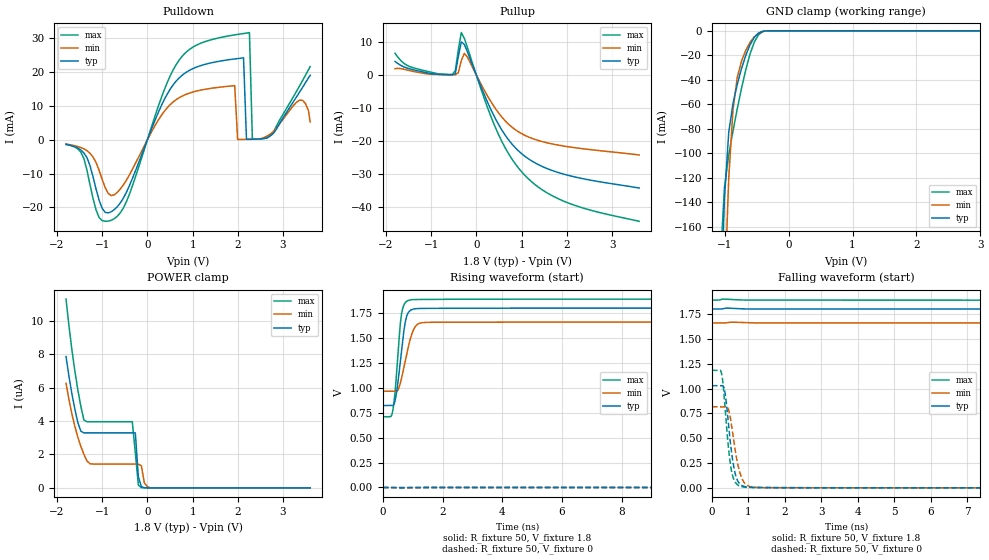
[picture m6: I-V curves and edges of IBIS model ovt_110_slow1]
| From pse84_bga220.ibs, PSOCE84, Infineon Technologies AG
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[Model] ovt_110_slow1
Model_type I/O
Enable   Active-High
Vinl  =  0.54
Vinh  =  1.26
Vmeas =  0.9
Cref  =  15e-12
| Capacitance   typ   min   max
C_comp   1.39974e-12   1.35992e-12   1.44753e-12
| Variables   typ   min   max
[GND Clamp Reference]   0   0   0
[POWER Clamp Reference]   1.8   1.66   1.89
[Pulldown Reference]   0   0   0
[Pullup Reference]   1.8   1.66   1.89
[Temperature Range]   25   125   -40
[Voltage Range]   1.8   1.66   1.89
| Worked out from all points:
|   slope of the pulldown table from 0 to 0.27 V, typ, clamps not added: 30.3 ohm
|   slope of the pullup table from 0 to 0.27 V, typ, clamps not added: 30.5 ohm
|   GND clamp passes 1 mA (typ) near -0.43 V on its own axis
|   falling waveform, R_fixture 50, V_fixture 1.8: 20-80 % time 92.1ns typ, 146ns min, 49.7ns max; typ from 1.8 V to 0.822 V
|   falling waveform, R_fixture 50, V_fixture 0: 20-80 % time 197ps typ, 231ps min, 178ps max; typ from 1.03 V to 0 V
|   rising waveform, R_fixture 50, V_fixture 1.8: 20-80 % time 231ps typ, 319ps min, 184ps max; typ from 0.822 V to 1.8 V
|   rising waveform, R_fixture 50, V_fixture 0: 20-80 % time 107ns typ, 168ns min, 63.3ns max; typ from 0 V to 1.03 V
[GND Clamp]
| Voltage   I(typ)   I(min)   I(max)
-1.271V   -717.5mA   -832.8mA   -643.6mA
-1.07V    -241.9mA   -348.3mA   -192.2mA
-1.003V   -137.2mA   -218.1mA   -128.1mA
-936.6mV  -83.06mA   -120.7mA   -101.3mA
-869.7mV  -59.26mA   -64.32mA   -81.77mA
-802.8mV  -43.7mA    -38.08mA   -63.69mA
-735.9mV  -30.76mA   -24.63mA   -46.83mA
-602.1mV  -11.27mA   -9.362mA   -18.72mA
-535.2mV  -5.241mA   -4.803mA   -9.042mA
-468.3mV  -1.746mA   -1.965mA   -3.086mA
-334.5mV  -35.9uA    -120.8uA   -33.39uA
3.6V      0A         0A         0A
[POWER Clamp]
| Voltage   I(typ)   I(min)   I(max)
-1.8V     7.872uA    6.273uA    11.31uA
-1.672V   5.671uA    4.461uA    8.32uA
-1.539V   3.91uA     3.037uA    5.87uA
-1.405V   3.295uA    2.008uA    4.063uA
-1.271V   3.295uA    1.447uA    3.964uA
-334.5mV  3.295uA    1.429uA    3.964uA
-267.6mV  3.295uA    1.429uA    2.099uA
-200.7mV  664.1nA    1.429uA    166.6nA
-133.8mV  69.92nA    1.319uA    14.86nA
-66.9mV   7.33nA     291.5nA    4.066nA
62.07mV   0A         0A         0A
3.6V      0A         0A         0A
[Pulldown]
| Voltage   I(typ)   I(min)   I(max)
-1.8V     -1.438mA   -1.35mA    -1.317mA
-1.405V   -3.903mA   -2.719mA   -5.566mA
-802.8mV  -21.26mA   -16.48mA   -23.79mA
931mV     20.46mA    13.74mA    26.61mA
1.93V     23.81mA    15.94mA    30.9mA
1.996V    23.92mA    60.76uA    31.04mA
2.126V    24.14mA    87.8uA     31.3mA
2.191V    90.18uA    111.8uA    31.42mA
2.256V    101.7uA    127.7uA    31.58mA
2.321V    127.9uA    151.7uA    138.4uA
3.364V    14.01mA    11.64mA    15.82mA
3.6V      18.99mA    5.217mA    21.55mA
[Pullup]
| Voltage   I(typ)   I(min)   I(max)
-1.8V     4.194mA    2.014mA    6.66mA
-1.472V   1.939mA    1.399mA    2.629mA
-535.2mV  164.9uA    119.7uA    248uA
-468.3mV  454.7uA    163.9uA    1.343mA
-401.4mV  5.638mA    785.3uA    7.615mA
-334.5mV  10.09mA    4.454mA    12.94mA
-267.6mV  9.357mA    6.64mA     11.17mA
-200.7mV  7.133mA    5.534mA    8.452mA
434.5mV   -13.51mA   -10.36mA   -16.28mA
1.055V    -24.34mA   -18.07mA   -30.05mA
1.996V    -30.17mA   -21.56mA   -38.47mA
3.6V      -34.13mA   -24.13mA   -44.2mA
[Ramp]
dV/dt_r   0.617141/0.107374u  0.488479/0.167637u  0.709896/63.2601n
dV/dt_f   0.586708/92.0937n  0.416414/0.145951u  0.708161/49.6813n
R_load = 50
[Falling Waveform]
R_fixture = 50
V_fixture = 1.8
V_fixture_min = 1.66
V_fixture_max = 1.89
| Time   V(typ)   V(min)   V(max)
0s        1.8V       1.66V      1.89V
11ns      1.8V       1.66V      1.864V
21.21ns   1.766V     1.658V     1.662V
39.28ns   1.599V     1.615V     1.317V
64.35ns   1.373V     1.509V     1.002V
89.43ns   1.199V     1.403V     840.8mV
122.9ns   1.044V     1.285V     756.7mV
195.1ns   891.7mV    1.123V     716.5mV
318.1ns   832.8mV    1.013V     710mV
800ns     822.2mV    966mV      709.7mV
[Falling Waveform]
R_fixture = 50
V_fixture = 0
V_fixture_min = 0
V_fixture_max = 0
| Time   V(typ)   V(min)   V(max)
0s        1.029V     816mV      1.183V
268.7ps   1.029V     816mV      1.146V
364.9ps   947.2mV    816mV      792.5mV
440.3ps   698.5mV    802.8mV    459.5mV
498.8ps   484.7mV    721.5mV    264.3mV
630ps     158.6mV    400.7mV    63.73mV
784.8ps   33.41mV    133.7mV    14.64mV
930.6ps   9.715mV    34.71mV    5.985mV
2.004ns   1.809mV    1.626mV    1.559mV
800ns     18.69nV    975.7nV    8.58nV
[Rising Waveform]
R_fixture = 50
V_fixture = 1.8
V_fixture_min = 1.66
V_fixture_max = 1.89
| Time   V(typ)   V(min)   V(max)
0s        822.1mV    965.5mV    709.7mV
260.9ps   822.3mV    965.5mV    710.7mV
332ps     822.3mV    965.6mV    769.1mV
443.9ps   925.7mV    965.4mV    1.081V
594.4ps   1.29V      1.058V     1.668V
719.4ps   1.604V     1.226V     1.841V
846.7ps   1.752V     1.404V     1.876V
1.097ns   1.794V     1.619V     1.886V
2.016ns   1.798V     1.658V     1.888V
800ns     1.8V       1.66V      1.89V
[Rising Waveform]
R_fixture = 50
V_fixture = 0
V_fixture_min = 0
V_fixture_max = 0
| Time   V(typ)   V(min)   V(max)
0s        18.59nV    971.3nV    8.569nV
15.69ns   247.9uV    88.48uV    22.41mV
27.55ns   36.21mV    4.594mV    196mV
54.29ns   251.5mV    81.06mV    600mV
81.31ns   462.9mV    197.6mV    870.2mV
106.4ns   620.1mV    302.1mV    1.01V
148.2ns   798.5mV    449.2mV    1.112V
224.5ns   945.7mV    626mV      1.166V
344.6ns   1.009V     747.9mV    1.181V
800ns     1.029V     814.1mV    1.183V
